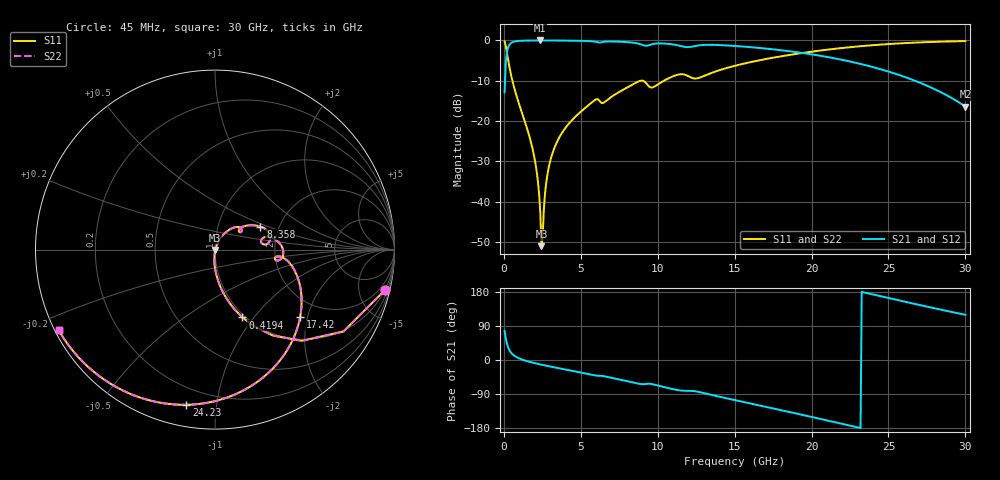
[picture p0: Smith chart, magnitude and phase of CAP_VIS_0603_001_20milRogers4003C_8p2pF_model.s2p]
! S-parameter model data by Modelithics Inc.  support@modelithics.com  813-866-6335  Tampa FL USA
! S-Parameter data specifications:
! Substrate: 20-mil Rogers 4003C, substrate thickness, H=0.508mm, Dielectric constant, Er=3.75
! PCB Mounting Pad Footprint: Pad width, PadW=0.90mm , Pad length, PadL=1.00mm , Pad gap, PadG (edge-to-edge)=1.00mm , Reference planes=3.0mm apart
! Created Wed Nov 18 13:25:11 2015
# hz S ma R 50
! 2 Port Network Data from SP1.SP block
! freq  magS11  angS11  magS21  angS21  magS12  angS12  magS22  angS22
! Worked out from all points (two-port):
!   401 points, 45 MHz to 30 GHz, reference 50 ohm
!   highest |S21| = -0.02 dB at 2.367 GHz (marker M1); lowest = -16.4 dB at 30 GHz (marker M2)
!   |S21| within 3 dB of the highest: 192.6 MHz to 19.21 GHz (19.02 GHz wide, 196 % of centre)
!   lowest |S11| = -51.0 dB at 2.441 GHz (marker M3), VSWR 1.01, Z = 50.2 - j0.236 ohm
!   |S11| at or under -10 dB: 550.5 MHz to 8.911 GHz (8.361 GHz wide, 177 % of centre); 9.01 GHz to 10.4 GHz (1.393 GHz wide, 14.4 % of centre)
!   |S22| runs from -51.0 to -0.2 dB; largest |S21 - S12| = 0
!   S11 on the Smith chart (normalised r, x): 45 MHz: 0.97, -8.42; 419.4 MHz: 0.97, -0.88; 8.358 GHz: 1.60, +0.45; 17.42 GHz: 1.51, -1.80; 24.23 GHz: 0.11, -0.83; 30 GHz: 0.01, -0.24
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4.5e7  0.9738 -13.4  0.2273 76.6  0.2273 76.6  0.9738 -13.4
2.696625e8  0.5769 -56.1  0.8162 33.9  0.8162 33.9  0.5769 -56.1
4.194375e8  0.4076 -68.0  0.9123 21.9  0.9123 21.9  0.4076 -68.0
8.687625e8  0.1912 -83.1  0.9803 6.6  0.9803 6.6  0.1912 -83.1
1.917188e9  0.04051 -95.0  0.9972 -7.5  0.9972 -7.5  0.04051 -95.0
2.14185e9  0.02281 -94.9  0.9977 -9.6  0.9977 -9.6  0.02281 -94.9
2.366512e9  0.007188 -85.8  0.9978 -11.7  0.9978 -11.7  0.007188 -85.8
2.4414e9  0.002809 -56.8  0.9978 -12.3  0.9978 -12.3  0.002809 -56.8
2.591175e9  0.007793 60.9  0.9977 -13.6  0.9977 -13.6  0.007793 60.9
2.74095e9  0.01667 67.7  0.9975 -14.9  0.9975 -14.9  0.01667 67.7
2.890725e9  0.02527 68.8  0.9972 -16.2  0.9972 -16.2  0.02527 68.8
3.265162e9  0.04555 67.8  0.9963 -19.3  0.9963 -19.3  0.04555 67.8
3.93915e9  0.07926 63.4  0.9938 -24.6  0.9938 -24.6  0.07926 63.4
5.062462e9  0.1337 54.7  0.9864 -33.5  0.9864 -33.5  0.1337 54.7
8.357512e9  0.2833 27.0  0.9385 -59.0  0.9385 -59.0  0.2833 27.0
1.007992e10  0.2902 14.0  0.917 -68.1  0.917 -68.1  0.2902 14.0
1.50225e10  0.4846 -18.4  0.8527 -106.0  0.8527 -106.0  0.4846 -18.4
1.74189e10  0.606 -38.6  0.7777 -127.1  0.7777 -127.1  0.606 -38.6
2.003996e10  0.726 -61.8  0.6695 -150.6  0.6695 -150.6  0.726 -61.8
2.423366e10  0.8794 -100.5  0.4531 170.7  0.4531 170.7  0.8794 -100.5
2.505742e10  0.9018 -108.2  0.4075 163.1  0.4075 163.1  0.9018 -108.2
3e10  0.9802 -152.7  0.1511 119.2  0.1511 119.2  0.9802 -152.7
